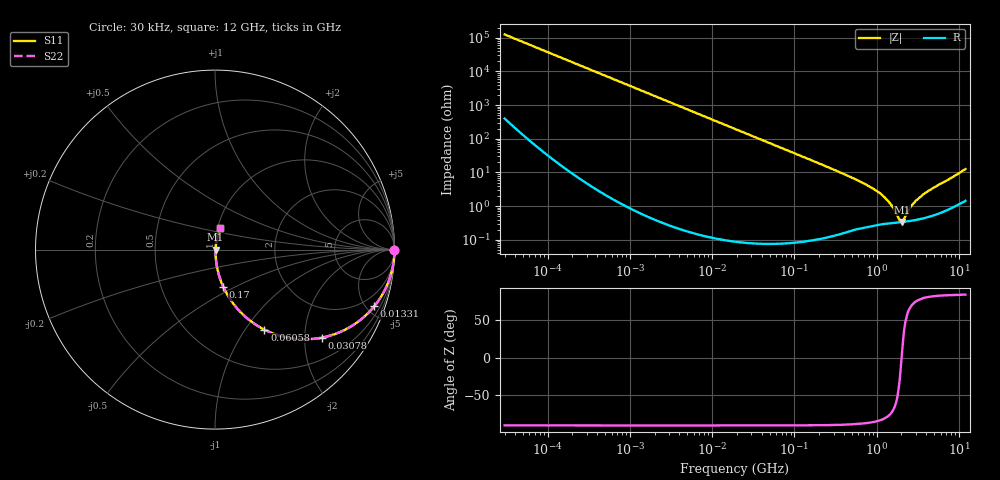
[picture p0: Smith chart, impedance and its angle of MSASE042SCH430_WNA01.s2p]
! MSASE042SCH430_WNA01  S-PARAMETER MODEL  ( General Type )
! Model Generated by TAIYO YUDEN Corporation (http://www.ty-top.com)
! Version 2.0
! TAIYO YUDEN Control No. 131101
! Copyright(c) 2012 TAIYO YUDEN CO.,LTD. All Rights Reserved.
! Product Description (link to TY-COMPAS)
! https://ds.yuden.co.jp/TYCOMPAS/or/detail?pn=MSASE042SCH430JWNA01&u=M
! Products Name : Multilayer Ceramic Capacitors
! Characteristics :
!  Capacitance : 43 pF , Rated Voltage : 16V , TCC : CH / C0H
!  Case Size : 0.4 x 0.2 / 0.016 x 0.008 [mm/inch] , Thickness : 0.2 / 0.008 [mm/inch]
!  (Conditions: Temperature = 25 degC , DC Bias Current/Voltage = 0A / 0V)
! External Node Assignments :
!  1  o---| |---o  2
! GND o---------o GND
! Frequency Range : 0.03MHz  -  12000MHz  [ 401 STEP ]
# MHz S RI R 50
! Freq[MHz].  S11 Real  S11 Imag  S21 Real  S21 Imag  S12 Real  S12 Imag  S22 Real  S22 Imag
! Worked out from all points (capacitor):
!   401 points, 30 kHz to 12 GHz, reference 50 ohm
!   read as one part in series: C = 42.6 pF near 32 kHz
!   lowest |Z| = 339 mohm at 2.037 GHz (marker M1)
!   series resonance near 2.01 GHz, so ESL is about 150 pH
!   S11 on the Smith chart (normalised r, x): 30 kHz: open; 13.31 MHz: 1.00, -5.61; 30.78 MHz: 1.00, -2.43; 60.58 MHz: 1.00, -1.23; 170 MHz: 1.00, -0.44; 12 GHz: 1.03, +0.25
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0.03  1 -0.000803  3.21e-06 0.000803  3.21e-06 0.000803  1 -0.000803
0.260295  0.9999 -0.00697  5.14e-05 0.00697  5.14e-05 0.00697  0.9999 -0.00697
2.258455  0.9963 -0.0602  0.00366 0.0602  0.00366 0.0602  0.9963 -0.0602
5.753879  0.9768 -0.1505  0.0232 0.1505  0.0232 0.1505  0.9768 -0.1505
13.30744  0.8873 -0.3161  0.1127 0.3161  0.1127 0.3161  0.8873 -0.3161
18.97367  0.7947 -0.4037  0.2053 0.4037  0.2053 0.4037  0.7947 -0.4037
30.77716  0.5954 -0.4905  0.4046 0.4905  0.4046 0.4905  0.5954 -0.4905
42.48934  0.4357 -0.4954  0.5643 0.4954  0.5643 0.4954  0.4357 -0.4954
60.58103  0.2753 -0.4461  0.7247 0.4461  0.7247 0.4461  0.2753 -0.4461
95.14999  0.1335 -0.3391  0.8665 0.3391  0.8665 0.3391  0.1335 -0.3391
164.6252  0.0492 -0.2141  0.9508 0.2141  0.9508 0.2141  0.0492 -0.2141
170.0206  0.0463 -0.2078  0.9537 0.2078  0.9537 0.2078  0.0463 -0.2078
749.4426  0.00417 -0.0427  0.9958 0.0427  0.9958 0.0427  0.00417 -0.0427
1103.571  0.0034 -0.0236  0.9966 0.0236  0.9966 0.0236  0.0034 -0.0236
1428.372  0.0032 -0.0123  0.9968 0.0123  0.9968 0.0123  0.0032 -0.0123
1625.032  0.00321 -0.00756  0.9968 0.00756  0.9968 0.00756  0.00321 -0.00756
1909.359  0.00329 -0.00184  0.9967 0.00184  0.9967 0.00184  0.00329 -0.00184
2036.564  0.00335 0.00045  0.9967 -0.00045  0.9967 -0.00045  0.00335 0.00045
2172.242  0.00342 0.00272  0.9966 -0.00272  0.9966 -0.00272  0.00342 0.00272
2722.352  0.00382 0.0103  0.9962 -0.0103  0.9962 -0.0103  0.00382 0.0103
3639.072  0.00473 0.0212  0.9953 -0.0212  0.9953 -0.0212  0.00473 0.0212
12000  0.0289 0.1195  0.9711 -0.1195  0.9711 -0.1195  0.0289 0.1195
